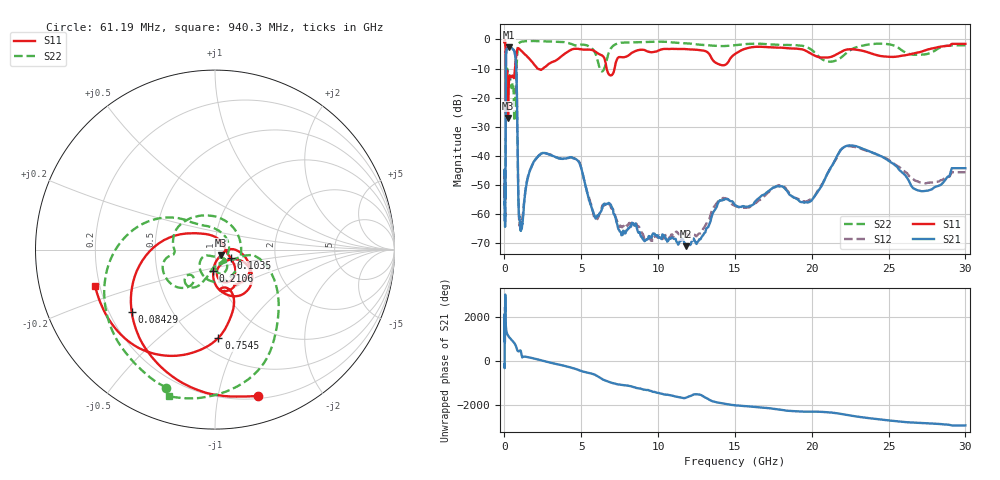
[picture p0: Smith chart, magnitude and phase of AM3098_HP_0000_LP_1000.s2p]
! Date/Time: Thu, Feb 28, 2019 8:30 AM
! Network Analyzer: Agilent Technologies E8364B Rev: A.07.50.67
! Sweep from 0.010 to 30.000 GHz, 1601 Points, Sweep Type: LOG
! Power Supply: 5.023 V, 0.002 A
# Hz S DB R 50
!freq MagS11 AngS11 MagS21 AngS21 MagS12 AngS12 MagS22 AngS22
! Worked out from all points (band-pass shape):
!   1601 points, 10 MHz to 30 GHz, reference 50 ohm
!   highest |S21| = -2.72 dB at 266.5 MHz (marker M1); lowest = -71.0 dB at 11.83 GHz (marker M2)
!   |S21| within 3 dB of the highest: 104.6 MHz to 705.4 MHz (600.8 MHz wide, 148 % of centre)
!   lowest |S11| = -26.9 dB at 233.9 MHz (marker M3), VSWR 1.09, Z = 53.3 - j3.27 ohm
!   |S11| at or under -10 dB: 90.38 MHz to 682.4 MHz (592 MHz wide, 153 % of centre); 2.161 GHz to 2.515 GHz (353.9 MHz wide, 15.1 % of centre); 6.649 GHz to 7.167 GHz (518.2 MHz wide, 7.5 % of centre)
!   |S22| runs from -28.1 to -0.5 dB; largest |S21 - S12| = 0.011
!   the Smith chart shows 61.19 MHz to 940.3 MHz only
!   S11 on the Smith chart (normalised r, x): 61.19 MHz: 0.22, -1.31; 84.29 MHz: 0.29, -0.31; 103.5 MHz: 1.19, -0.11; 210.6 MHz: 0.95, -0.23; 754.5 MHz: 0.63, -0.82; 940.3 MHz: 0.18, -0.15
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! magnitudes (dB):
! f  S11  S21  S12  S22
! 10 MHz  -0.4  -46.3  -49.2  -0.6
! 38.04 MHz  -0.5  -60.8  -60.4  -1.0
! 61.19 MHz  -1.4  -52.0  -53.2  -1.8
! 71.46 MHz  -2.0  -50.4  -51.4  -2.5
! 84.29 MHz  -4.7  -27.6  -27.4  -5.2
! 95.05 MHz  -21.1  -9.8  -9.8  -22.1
! 103.5 MHz  -20.0  -5.9  -5.9  -14.8
! 144.7 MHz  -14.6  -3.4  -3.3  -12.7
! 210.6 MHz  -18.3  -2.9  -2.9  -11.7
! 233.9 MHz  -26.9  -2.8  -2.8  -12.6
! 266.5 MHz  -17.6  -2.7  -2.7  -13.0
! 550.5 MHz  -12.6  -3.4  -3.4  -14.9
! 639.6 MHz  -12.7  -4.1  -4.0  -28.1
! 754.5 MHz  -6.2  -8.7  -8.7  -19.4
! 940.3 MHz  -3.1  -60.3  -59.9  -1.3
! 2.084 GHz  -9.6  -40.8  -40.7  -0.6
! 4.687 GHz  -3.2  -41.2  -41.1  -2.1
! 7.926 GHz  -5.9  -65.6  -64.0  -1.0
! 11.83 GHz  -3.4  -71.0  -66.7  -1.4
! 19.7 GHz  -4.2  -56.0  -55.5  -2.7
! 22.56 GHz  -3.4  -36.4  -36.7  -3.5
! 30 GHz  -1.5  -44.2  -45.6  -2.0
